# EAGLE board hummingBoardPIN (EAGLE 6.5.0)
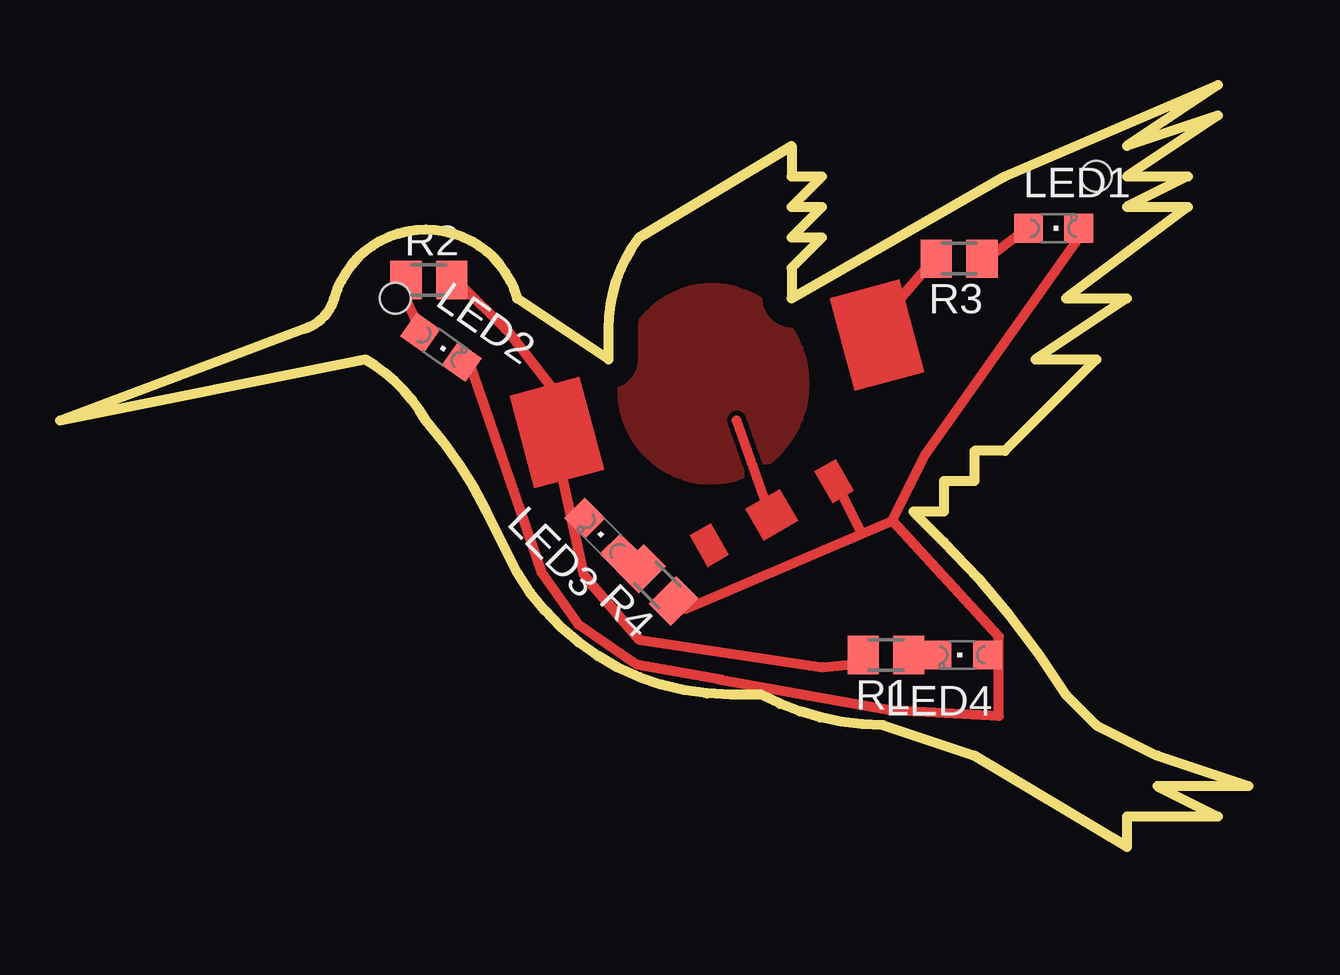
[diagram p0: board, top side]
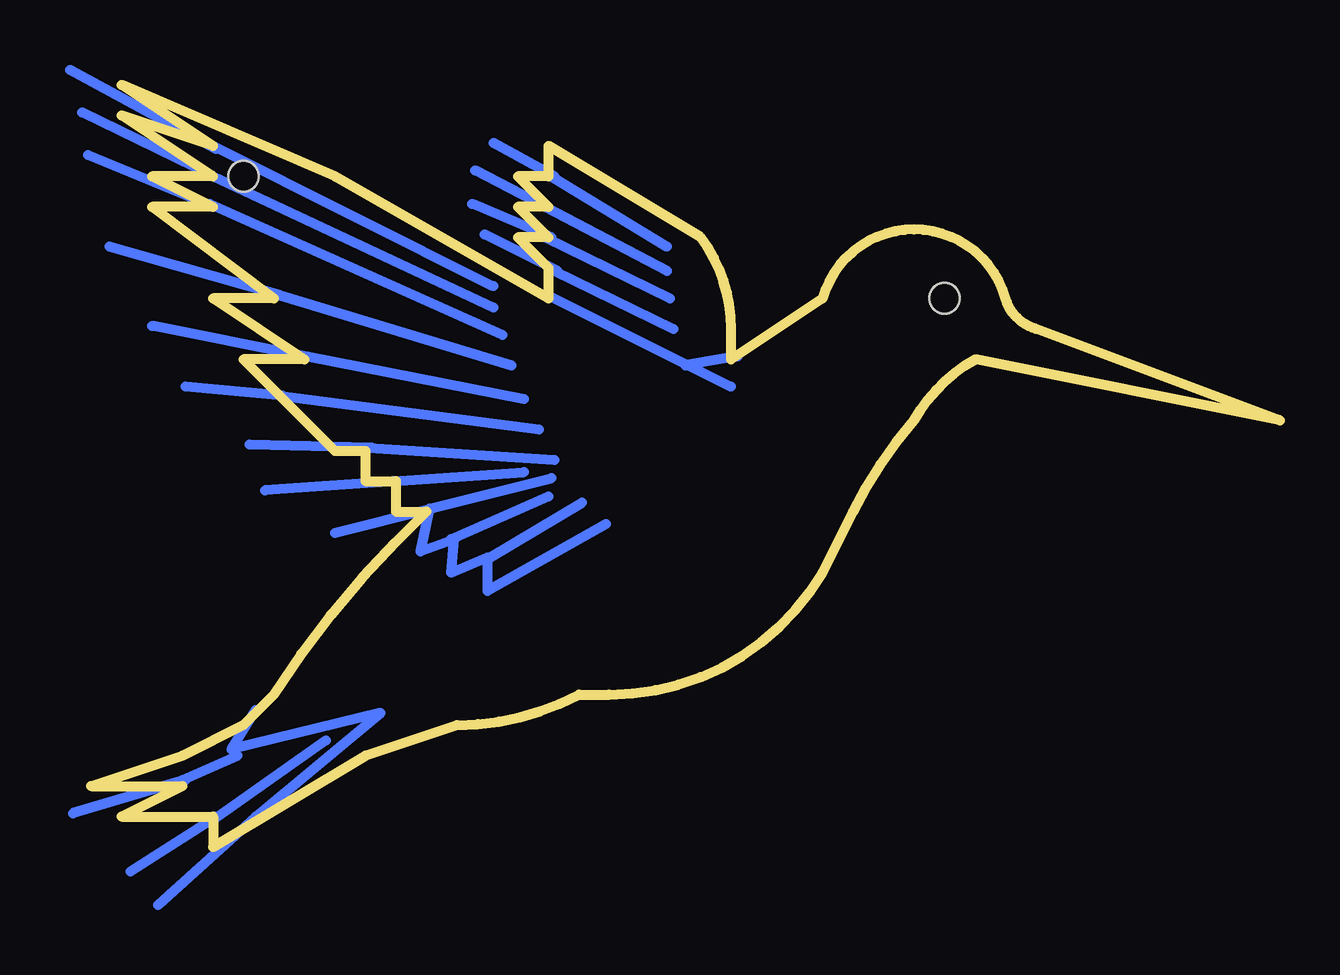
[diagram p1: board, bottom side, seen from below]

Size 49.53 x 31.75 mm. Coordinates in mm from the lower left corner, seen from the top.
Outline: 0,17.78 10.16,21.59 arc58 11.43,22.86 arc-148 19.05,22.86 22.86,20.32 22.86,21.59 arc-37 24.13,25.4 30.48,29.21 30.48,27.94 31.75,27.94 30.48,26.67 31.75,26.67 30.48,25.4 31.75,25.4 30.48,24.13 30.48,22.86 39.37,27.94 48.26,31.75 44.45,29.21 48.26,30.48 44.45,27.94 46.99,27.94 44.45,26.67 46.99,26.67 41.91,22.86 44.45,22.86 40.64,20.32 43.18,20.32 39.37,16.51 38.1,16.51 38.1,15.24 36.83,15.24 36.83,13.97 35.56,13.97 36.83,12.7 arc-13 41.91,6.35 43.18,5.08 45.72,3.81 49.53,2.54 45.72,2.54 48.26,1.27 44.45,1.27 44.45,0 38.1,3.81 34.29,5.08 arc-28 29.21,6.35 27.94,6.35 arc-59 19.05,11.43 17.78,13.97 arc14 15.24,17.78 arc31 12.7,20.32 0,17.78
Copper layers (1*16): Top 0.035mm / dielectric 1.5mm / Bottom 0.035mm
Design rules "default": minimum track width 10mil, minimum drill 24mil, track to track 8mil, track to pad 8mil, pad to pad 8mil, via to via 8mil, smd to smd 8mil, copper to edge 40mil, drill to drill 8mil, minimum pad ring 10mil, minimum via ring 8mil, stop-mask expansion 4mil, vias tented up to drill 0mil, thermal gap 10mil
Holes 1.27 mm at 13.97,22.86 43.18,27.94

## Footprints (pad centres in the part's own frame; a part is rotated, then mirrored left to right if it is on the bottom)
CHIPLED_0805 = smd 1.2 x 1.2: A 0,-1.05; C 0,1.05
M0805 = smd 1.3 x 1.6: 1 -0.95,0; 2 0.95,0

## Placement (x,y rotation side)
LED1  [CHIPLED_0805]  41.4,25.78 270 top
LED2  [CHIPLED_0805]  15.88,20.83 235 top
LED3  [CHIPLED_0805]  22.61,12.95 45 top
LED4  [CHIPLED_0805]  37.59,8 90 top
R1  [M0805]  34.42,8 180 top
R2  [M0805]  15.37,23.62 0 top
R3  [M0805]  37.47,24.51 180 top
R4  [M0805]  24.89,10.92 135 top

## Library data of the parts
LED1-LED4 = led
R1-R4 = resistor

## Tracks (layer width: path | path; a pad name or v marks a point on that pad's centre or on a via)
N$10
  Bottom 0.406: 30.48,22.99 22.86,19.18
N$11
  Bottom 0.406: 22.61,20.45 24.77,20.07
N$12
  Bottom 0.406: 42.67,5.71 43.69,4.06 37.47,5.59 42.67,1.27 46.74,-2.41
N$13
  Bottom 0.406: 44.45,1.14 39.75,4.45
N$14
  Bottom 0.406: 45.72,2.79 43.43,3.81
N$15
  Bottom 0.406: 30.35,27.94 25.53,25.02
N$16
  Bottom 0.406: 25.53,24 30.61,26.67 33.53,28.19
N$17
  Bottom 0.406: 30.61,25.4 25.4,22.86
N$18
  Bottom 0.406: 30.23,24 25.27,21.59
N$19
  Bottom 0.406: 44.45,29.21 32.77,23.37
N$20
  Bottom 0.406: 32.77,22.48 44.45,27.94 49.91,30.61
N$21
  Bottom 0.406: 44.58,26.8 32.38,21.34
N$22
  Bottom 0.406: 32,20.07 41.66,22.99 48.77,25.02
N$23
  Bottom 0.406: 40.51,20.45 31.5,18.67
N$24
  Bottom 0.406: 41.66,18.8 30.86,17.4
N$25
  Bottom 0.406: 37.97,16.64 30.23,16.13
N$26
  Bottom 0.406: 28.07,13.46 33.02,10.67 33.02,12.07 34.54,11.43 34.42,12.83 35.81,12.32 35.43,14.1 30.35,15.37
N$27
  Bottom 0.406: 32.89,12.07 29.08,14.35
N$28
  Bottom 0.406: 34.54,12.83 30.48,14.61
N$29
  Bottom 0.406: 36.96,15.24 31.5,15.62
N$30
  Bottom 0.406: 30.23,27.94 32.77,29.34
N$31
  Bottom 0.406: 30.35,25.4 33.66,26.8
N$32
  Bottom 0.406: 30.1,24 33.15,25.53
N$33
  Bottom 0.406: 44.32,29.08 50.42,32.39
N$34
  Bottom 0.406: 44.45,26.67 49.66,28.83
N$35
  Bottom 0.406: 40.64,20.45 46.99,21.72
N$36
  Bottom 0.406: 41.53,18.8 45.59,19.18
N$37
  Bottom 0.406: 37.85,16.64 42.93,16.76
N$38
  Bottom 0.406: 36.83,15.24 42.29,14.86
N$39
  Bottom 0.406: 35.31,14.1 39.37,13.08
N$40
  Bottom 0.406: 45.59,2.79 50.29,1.4
N$41
  Bottom 0.406: 44.32,1.27 47.88,-1.02
S$1
  pour Top: 31.04,19.3 arc90 27.04,23.3 arc90 23.42,19.18 arc90 27.04,15.3 arc90
S$2
  Top 0.406: 34.8,22.61 36.45,24.51
S$3
  Top 0.406: 38.61,24.51 40.13,25.65
S$4
  Top 0.406: 42.55,25.53 36.07,16.38
S$6
  Top 0.406: 31.75,7.49 33.02,7.62
S$7
  Top 0.406: 20.57,19.05 18.41,21.84
S$8
  Top 0.406: 31.75,7.49 24.13,8.64 21.84,11.3 20.7,16.51
S$9
  Top 0.406: 17.02,20.32 20.07,11.43 21.59,9.27 24,7.62 27.56,6.98
S$10
  Top 0.406: 18.54,21.59 16.76,23.37
S$11
  Top 0.406: 14.1,23.5 14.86,21.84
S$12
  Top 0.406: 27.43,6.98 34.54,5.71 39.12,5.46 39.12,8.76 34.67,13.59 | 34.67,13.59 36.07,16.38 | 26.04,9.91 34.67,13.59
S$14
  Top 0.406: 33.4,13.08 32.51,14.86
S$15
  Top 0.406: 29.59,13.84 28.19,17.78
(copper drawn outside any net)
  shapes: Bottom circle x1, Top area x5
